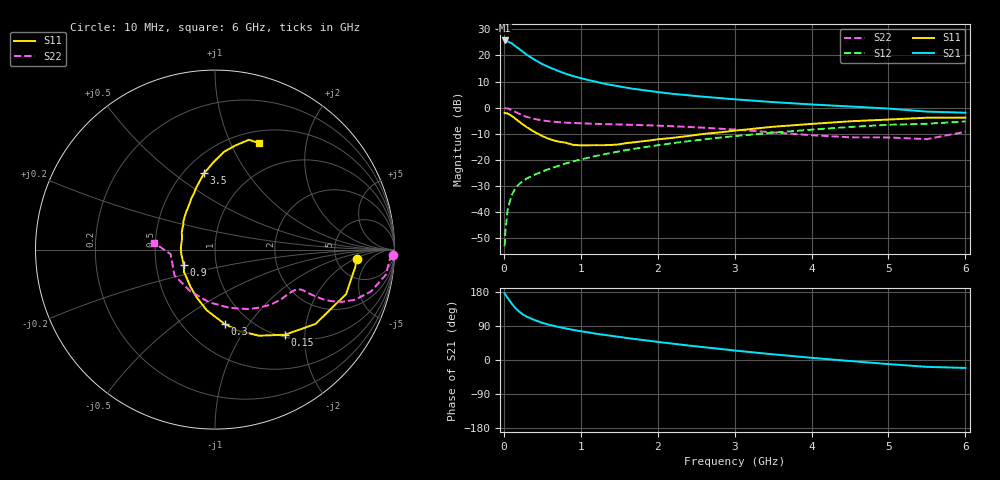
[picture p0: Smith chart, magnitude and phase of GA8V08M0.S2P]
! Infineon Technologies  Discrete & RF Semiconductors
! BF775
! Si NPN RF Bipolar Junction Transistor in SOT23
! VCE = 8 V  IC = 8 mA
! Common Emitter S-Parameters:  May  1996
# GHz  S  MA  R  50
!  f  S11  S21  S12  S22
! GHz  MAG  ANG  MAG  ANG  MAG  ANG  MAG  ANG
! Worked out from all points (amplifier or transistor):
!   36 points, 10 MHz to 6 GHz, reference 50 ohm
!   highest |S21| = 25.8 dB at 10 MHz (marker M1)
!   |S21| within 3 dB of that: start of sweep to 187.5 MHz
!   unconditionally stable (mu >= 1): 693.2 MHz to 2.92 GHz
!   at 250 MHz: K = 0.60, MSG = 24.7 dB, |S12| = -28.1 dB
!   at 1.4 GHz: K = 1.10, MAG = 11.1 dB, |S12| = -17.4 dB
!   at 6 GHz: K = 0.89, MSG = 1.7 dB, |S12| = -5.3 dB
!   S11 on the Smith chart (normalised r, x): 10 MHz: 8.00, -2.19; 150 MHz: 1.04, -1.59; 300 MHz: 0.77, -0.78; 900 MHz: 0.69, -0.12; 3.5 GHz: 0.62, +0.65; 6 GHz: 0.63, +1.29
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0.01  0.7918 -3.7  19.42 176.2  0.0022 87.9  0.9908 -1.6
0.02  0.7866 -7.5  19.07 172.8  0.0041 89.0  0.9746 -3.4
0.05  0.771 -18.8  18.61 163.7  0.0111 79.7  0.9631 -8.3
0.1  0.6968 -36.4  17.18 149.4  0.0207 73.4  0.899 -15.1
0.15  0.6148 -50.5  15.09 137.0  0.0284 66.9  0.8268 -19.8
0.2  0.5382 -63.0  13.32 127.7  0.0342 64.7  0.7617 -22.5
0.25  0.4713 -73.8  11.7 119.9  0.0394 61.9  0.7051 -24.0
0.3  0.4192 -82.4  10.31 114.1  0.0439 62.1  0.6622 -24.7
0.4  0.341 -97.8  8.274 105.5  0.0516 61.6  0.6056 -25.0
0.5  0.2843 -111.3  6.839 98.0  0.0595 62.0  0.5673 -25.0
0.6  0.2468 -124.0  5.851 92.5  0.0678 62.8  0.5437 -24.8
0.7  0.2237 -134.5  5.098 87.7  0.0757 63.6  0.5282 -25.0
0.9  0.1932 -154.2  4.032 79.5  0.0931 63.6  0.5074 -25.9
1.1  0.1897 -174.6  3.379 72.8  0.1096 63.9  0.494 -27.7
1.3  0.1902 170.5  2.896 66.5  0.1275 63.4  0.4835 -29.7
1.6  0.2094 152.2  2.402 58.0  0.154 61.9  0.4695 -33.6
2.2  0.2636 127.6  1.835 43.0  0.2085 57.8  0.4395 -43.4
3  0.3613 106.8  1.445 25.0  0.2838 50.2  0.3796 -60.8
3.5  0.4293 98.2  1.276 15.0  0.3301 44.6  0.3347 -76.0
4.5  0.5466 84.8  1.051 -2.7  0.4259 32.4  0.2696 -120.9
5.5  0.6404 72.8  0.838 -18.1  0.491 17.3  0.2485 -174.2
6  0.6426 67.7  0.799 -20.9  0.5412 13.2  0.3434 173.5
